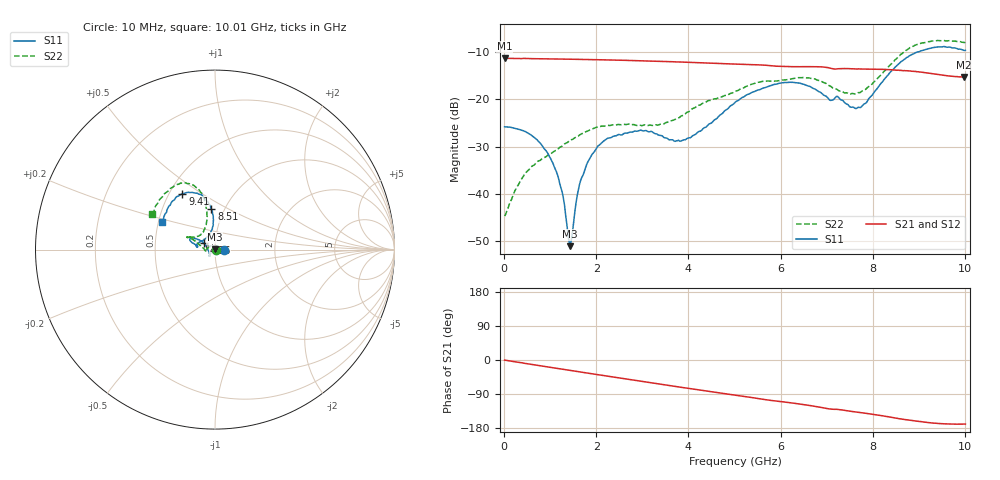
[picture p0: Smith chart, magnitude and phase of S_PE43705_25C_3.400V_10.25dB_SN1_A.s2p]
! Device ID: PE43705
! Serial: 1
! Insertion: A
! Impedance: 50 ohm
! Temp: 25C
! VDD: 3.400V
! Attenuation Step: 10.25dB
#  Hz  S  RI  R  50
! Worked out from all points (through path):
!   401 points, 10 MHz to 10.01 GHz, reference 50 ohm
!   highest |S21| = -11.26 dB at 10 MHz (marker M1); lowest = -15.2 dB at 9.985 GHz (marker M2)
!   group delay of S21, straight-line fit = 48.8 ps
!   lowest |S11| = -51.1 dB at 1.435 GHz (marker M3), VSWR 1.01, Z = 49.8 + j0.202 ohm
!   |S11| at or under -10 dB: start of sweep to 8.951 GHz
!   |S22| runs from -44.7 to -7.5 dB; largest |S21 - S12| = 0.0022
!   S11 on the Smith chart (normalised r, x): 10 MHz: 1.11, +0.00; 4.76 GHz: 0.88, +0.07; 8.51 GHz: 0.87, +0.41; 9.41 GHz: 0.58, +0.42; 10.01 GHz: 0.52, +0.18
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1e7  0.0514 4.99e-05  0.2734 -0.00129  0.2737 -0.00111  0.0058 0.000347
4.35e8  0.0447 0.0115  0.2693 -0.0407  0.2684 -0.0401  0.00261 0.0156
9.6e8  0.0221 0.014  0.2553 -0.0859  0.2554 -0.0858  -0.0153 0.0208
1.21e9  0.00924 0.00858  0.2463 -0.1059  0.2464 -0.1057  -0.0257 0.0176
1.385e9  0.000627 0.00366  0.2392 -0.1195  0.2393 -0.1195  -0.0324 0.0142
1.435e9  -0.00191 0.00203  0.2369 -0.1234  0.237 -0.1232  -0.0346 0.013
1.685e9  -0.013 -0.00728  0.2248 -0.1416  0.2249 -0.1415  -0.043 0.00632
1.885e9  -0.0206 -0.0142  0.2142 -0.1553  0.2143 -0.1551  -0.0483 0.001
2.21e9  -0.0267 -0.0266  0.1951 -0.1758  0.1952 -0.1757  -0.0523 -0.00704
2.935e9  -0.0308 -0.0354  0.1456 -0.2123  0.1459 -0.2123  -0.053 -0.00794
3.36e9  -0.0291 -0.0299  0.1139 -0.2265  0.1142 -0.2262  -0.0537 -0.00448
3.885e9  -0.0364 -0.00721  0.0735 -0.2376  0.0736 -0.2374  -0.067 0.00978
4.76e9  -0.0629 0.0373  0.00672 -0.2395  0.00709 -0.2395  -0.1007 0.0412
5.01e9  -0.0787 0.0495  -0.0115 -0.2367  -0.0113 -0.237  -0.112 0.0483
5.985e9  -0.1345 0.0642  -0.0749 -0.2116  -0.0739 -0.2117  -0.1429 0.0685
6.685e9  -0.127 0.0382  -0.1149 -0.1906  -0.1152 -0.1903  -0.1505 0.0691
7.685e9  -0.046 0.0687  -0.1566 -0.1414  -0.1562 -0.1415  -0.0683 0.0965
8.36e9  -0.0101 0.1895  -0.1799 -0.1025  -0.1792 -0.1029  -0.0473 0.2232
8.51e9  -0.0197 0.2244  -0.1827 -0.0908  -0.1818 -0.0917  -0.0556 0.2626
9.41e9  -0.1814 0.3118  -0.1799 -0.0402  -0.1795 -0.0398  -0.2195 0.3605
9.985e9  -0.288 0.1618  -0.17 -0.0322  -0.1702 -0.0327  -0.3431 0.2073
1.001e10  -0.2947 0.1533  -0.1706 -0.0329  -0.1708 -0.0333  -0.3508 0.1963
